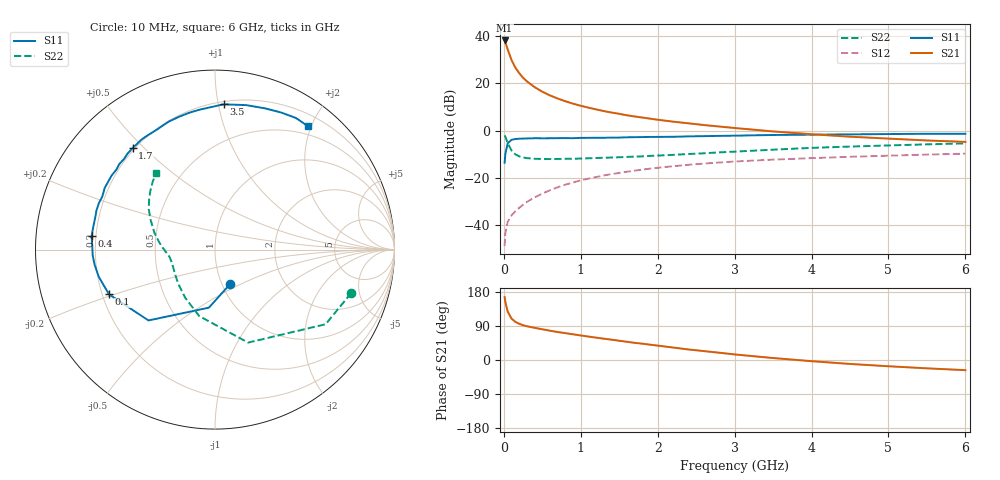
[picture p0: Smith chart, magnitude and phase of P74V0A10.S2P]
! SIEMENS Small Signal Semiconductors
! BFP196
! Si NPN RF Bipolar Junction Transistor in SOT143
! VCE = 4 V  IC = 100 mA
! Common Emitter S-Parameters:  May  1996
# GHz  S  MA  R  50
!  f  S11  S21  S12  S22
! GHz  MAG  ANG  MAG  ANG  MAG  ANG  MAG  ANG
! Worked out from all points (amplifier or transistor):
!   36 points, 10 MHz to 6 GHz, reference 50 ohm
!   highest |S21| = 38.2 dB at 10 MHz (marker M1)
!   |S21| within 3 dB of that: start of sweep to 42.14 MHz
!   unconditionally stable (mu >= 1): 334.2 MHz to 4.791 GHz
!   at 250 MHz: K = 0.94, MSG = 26.9 dB, |S12| = -31.4 dB
!   at 1.4 GHz: K = 1.09, MAG = 11.2 dB, |S12| = -18.4 dB
!   at 6 GHz: K = 0.98, MSG = 2.5 dB, |S12| = -9.7 dB
!   S11 on the Smith chart (normalised r, x): 10 MHz: 1.09, -0.44; 100 MHz: 0.23, -0.19; 400 MHz: 0.18, +0.05; 1.7 GHz: 0.19, +0.46; 3.5 GHz: 0.22, +1.04; 6 GHz: 0.37, +1.95
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0.01  0.2094 -66.2  81.15 166.0  0.0036 73.7  0.7966 -17.7
0.02  0.3252 -96.0  74.26 152.7  0.0068 66.0  0.7435 -34.0
0.05  0.5415 -133.2  52.45 127.7  0.0118 53.7  0.55 -70.4
0.1  0.6408 -157.1  31.2 109.2  0.0161 53.1  0.3802 -103.5
0.15  0.6654 -166.9  21.63 100.7  0.0198 55.0  0.3152 -121.8
0.2  0.6764 -173.1  16.48 95.5  0.0233 58.2  0.2861 -133.3
0.25  0.6825 -177.5  13.18 91.8  0.027 61.0  0.2708 -141.7
0.3  0.6833 179.1  11.06 89.1  0.0311 62.5  0.2625 -147.0
0.4  0.6916 173.8  8.354 84.9  0.0387 65.0  0.2545 -154.9
0.5  0.6901 169.8  6.681 81.1  0.0466 66.4  0.252 -159.8
0.6  0.6908 165.1  5.577 77.3  0.055 66.5  0.2513 -163.2
0.7  0.6955 161.7  4.795 73.8  0.0635 66.2  0.2522 -165.8
0.9  0.6941 154.7  3.728 67.8  0.0803 64.4  0.2548 -169.8
1.1  0.7054 147.4  3.069 61.8  0.0967 62.2  0.2607 -172.5
1.3  0.7076 140.9  2.6 56.2  0.113 59.3  0.2674 -175.1
1.7  0.7287 129.0  2 45.3  0.1427 53.6  0.2824 -180.0
2.2  0.743 115.7  1.553 32.9  0.1769 45.8  0.3078 173.9
2.8  0.7763 100.5  1.225 19.2  0.2122 36.6  0.3478 165.0
3.5  0.8109 86.6  0.965 5.2  0.2442 26.4  0.3964 155.0
4.5  0.8352 70.3  0.746 -10.4  0.2802 14.3  0.4613 142.7
5.5  0.8608 58.4  0.621 -22.0  0.312 3.5  0.5136 132.5
6  0.8608 53.0  0.579 -26.8  0.3265 -2.3  0.538 127.6
